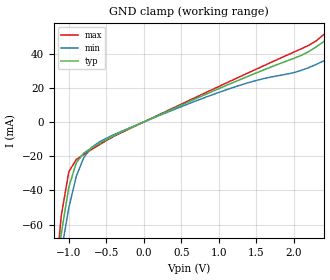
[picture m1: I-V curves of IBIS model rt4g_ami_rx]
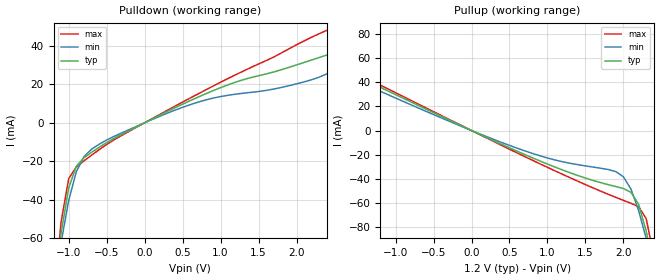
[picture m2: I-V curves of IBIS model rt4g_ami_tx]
|   Microsemi Corporation
|   RTG4 IBIS-AMI Models
[IBIS ver]   5.0
[File name]   rt4g_ami.ibs
[File Rev]   1.1
[Date]   Feb 16, 2018
[Disclaimer] These IBIS Models are Provided "As is" with NO WARRANTY
   whatsoever and signal integrity software specifically disclaims any
   implied warranties of merchantability, fitness for a particular
   purpose or against infringement.
[Notes] Known limitations: Main tap is limited to maximum amplitude setting only
   and cannot be adjusted
[Copyright]  (c) 2018, Microsemi Corporation, All Rights Reserved.
[Component]  RT4G_ibis_ami
[Manufacturer] Microsemi Corporation
[Package]
|   typ   min   max
| RT4G150
R_pkg   2.98   NA   NA   |150-CG1657
L_pkg   8.96nH   NA   NA   |150-CG1657
C_pkg   5.67pF   NA   NA   |150-CG1657
| RT4G150
|R_pkg   2.97   NA   NA   |150-LG1657
|L_pkg   8.11nH   NA   NA   |150-LG1657
|C_pkg   5.56pF   NA   NA   |150-LG1657
|RT4G150
|R_pkg   5.53   NA   NA   |150-CQ352
|L_pkg   23.11nH   NA   NA   |150-CQ352
|C_pkg   19.57pF   NA   NA   |150-CQ352
| The PIN numbers given below are examples. They do not correspond to
| device pin numbers.
[Pin]   signal_name   model_name   R_pin  L_pin  C_pin
1p   rt4g_tx_p   rt4g_ami_tx   NA   NA   NA
1n   rt4g_tx_n   rt4g_ami_tx   NA   NA   NA
2p   rt4g_rx_p   rt4g_ami_rx   NA   NA   NA
2n   rt4g_rx_n   rt4g_ami_rx   NA   NA   NA
[Diff_Pin] inv_pin vdiff tdelay_typ tdelay_min tdelay_max
1p   1n   0.1V  NA   NA   NA
2p   2n   0.1V  NA   NA   NA
| Models and submodels in the file (2): rt4g_ami_rx (Input), rt4g_ami_tx (Output)
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|   Model rt4g_ami_rx
[Model] rt4g_ami_rx
Model_type Input
C_comp 0.914p 0.471p 1.37p
Vinh = 0.55
Vinl = 0.45
[Algorithmic Model]
Executable Windows_VisualStudio7.1.3088_32 abicdr_rx.dll   abicdr_rx.ami
Executable Windows_VisualStudio7.1.3088_64 abicdr_x64_rx.dll   abicdr_rx.ami
Executable Linux_gcc3.2.3_64   abicdr_rh64_rx.dll  abicdr_rx.ami
[End Algorithmic Model]
[Temperature Range]   25C   125C   -55C
[Voltage Range]   1.2V   1.14V   1.26V
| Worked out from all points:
|   GND clamp passes 1 mA (typ) near -0.05 V on its own axis
[GND Clamp]
|Voltage   I(typ)   I(min)   I(max)
-2.5V     -710.8mA   -585.6mA   -919mA
-1.2V     -101.9mA   -106.1mA   -100.5mA
-1.1V     -65.27mA   -75.8mA    -54.63mA
-1V       -38.09mA   -50.18mA   -29.12mA
-900mV    -23.87mA   -31.72mA   -21.92mA
-800mV    -18.2mA    -20.83mA   -18.98mA
-700mV    -15.32mA   -15.03mA   -16.22mA
-600mV    -12.78mA   -11.88mA   -13.51mA
100mV     1.987mA    1.824mA    2.09mA
1V        19.46mA    17.27mA    20.72mA
2.2V      41.17mA    31.79mA    44.83mA
2.5V      50.17mA    37.82mA    55.2mA
|   Model rt4g_ami_tx
[Model] rt4g_ami_tx
Model_type Output
C_comp 0.914p 0.471p 1.37p
Cref = 0
Vref = 0.5
Rref = 50
Vmeas = 0.6
[Algorithmic Model]
Executable Windows_VisualStudio7.1.3088_32   abicdr_tx.dll   abicdr_tx.ami
Executable Windows_VisualStudio7.1.3088_64   abicdr_x64_tx.dll   abicdr_tx.ami
Executable Linux_gcc3.2.3_64   abicdr_rh64_tx.dll  abicdr_tx.ami
[End Algorithmic Model]
[Temperature Range]   25C   125C   -55C
[Voltage Range]   1.2V   1.14V   1.26V
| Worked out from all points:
|   slope of the pulldown table from 0 to 0.18 V, typ, clamps not added: 50.4 ohm
|   slope of the pullup table from 0 to 0.18 V, typ, clamps not added: 34.2 ohm
[Pulldown]
|Voltage   I(typ)   I(min)   I(max)
-2.5V     -663.6mA   -535.6mA   -873.7mA
-1.2V     -90.34mA   -89.14mA   -93.67mA
-1.1V     -57.52mA   -62.43mA   -51.53mA
-1V       -33.95mA   -40.47mA   -29.14mA
-900mV    -22.69mA   -25.54mA   -23.01mA
-800mV    -18.27mA   -17.71mA   -19.89mA
-600mV    -12.82mA   -11.22mA   -14.05mA
100mV     1.995mA    1.723mA    2.182mA
700mV     13.31mA    10.7mA     14.97mA
1.2V      21.19mA    14.92mA    25.04mA
1.9V      28.88mA    19.31mA    38.53mA
2.5V      36.63mA    27.48mA    49.9mA
[Pullup]
|Voltage   I(typ)   I(min)   I(max)
-3.7V     173.4mA    162.2mA    188.3mA
-2.7V     88.71mA    88.6mA     87.4mA
-1.9V     57.14mA    53.33mA    59.63mA
-100mV    2.954mA    2.608mA    3.146mA
1V        -27.86mA   -22.82mA   -30.6mA
1.9V      -46.55mA   -34.12mA   -55.56mA
2V        -48.22mA   -38.42mA   -58.05mA
2.1V      -51.37mA   -48.68mA   -60.46mA
2.2V      -61.31mA   -66.37mA   -63.34mA
2.3V      -83.51mA   -89.64mA   -73.16mA
2.4V      -114.9mA   -116.4mA   -103.7mA
3.6V      -622.5mA   -520.6mA   -796mA
[Ramp]
| variable   typ   min   max
dV/dt_r 0.3912/8.652e-11   0.3423/9.022e-11   0.4256/9.625e-11
dV/dt_f 0.3912/7.387e-11   0.3423/7.781e-11   0.4256/7.198e-11
R_load = 50
|End [Model] rt4g_ami_tx
|End [Component]
